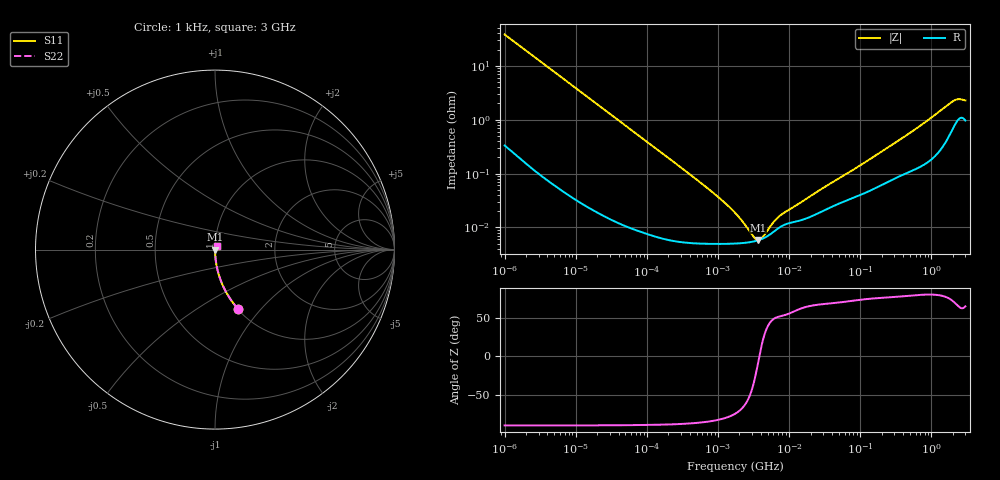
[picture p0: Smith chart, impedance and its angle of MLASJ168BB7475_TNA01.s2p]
! MLASJ168BB7475_TNA01  S-PARAMETER MODEL  ( Standard Model )
! Model Generated by TAIYO YUDEN Corporation (http://www.ty-top.com)
! Version 1.0
! TAIYO YUDEN Control No. 220601
! Copyright(c) 2014 TAIYO YUDEN CO.,LTD. All Rights Reserved.
! Product Description (link to TY-COMPAS)
! https://ds.yuden.co.jp/TYCOMPAS/or/detail?pn=MLASJ168BB7475KTNA01&u=M
! Products Name : Multilayer Ceramic Capacitors
! Characteristics :
!  Capacitance : 4.7 [uF] , Rated Voltage : 6.3 [V] , TCC : X7R
!  Case Size : 1.6 x 0.8 / 0.063 x 0.031 [mm/inch] , Thickness : 0.8 / 0.031 [mm/inch]
!  (Conditions: Temperature = 25 [degC] , DC Bias Voltage = 0 [V])
! External Node Assignments :
!  1  o---| |---o  2
! GND o---------o GND
! Frequency Range : 1kHz  -  3GHz  [ 401 STEP ]
# MHZ S RI R 50
! Freq[MHz].  S11 Real  S11 Imag  S21 Real  S21 Imag  S12 Real  S12 Imag  S22 Real  S22 Imag
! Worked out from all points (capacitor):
!   401 points, 1 kHz to 3 GHz, reference 50 ohm
!   read as one part in series: C = 4.16 uF near 1.077 kHz
!   lowest |Z| = 5.82 mohm at 3.651 MHz (marker M1)
!   series resonance near 3.805 MHz, so ESL is about 420 pH
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0.001  0.1293 -0.3313  0.8707 0.3313  0.8707 0.3313  0.1293 -0.3313
0.001685  0.0507 -0.2153  0.9493 0.2153  0.9493 0.2153  0.0507 -0.2153
0.00306  0.0164 -0.1233  0.9836 0.1233  0.9836 0.1233  0.0164 -0.1233
0.005768  0.00495 -0.0664  0.995 0.0664  0.995 0.0664  0.00495 -0.0664
0.01216  0.00128 -0.0317  0.9987 0.0317  0.9987 0.0317  0.00128 -0.0317
0.147855  7.14e-05 -0.00264  0.9999 0.00264  0.9999 0.00264  7.14e-05 -0.00264
0.791611  4.97e-05 -0.000475  1 0.000475  1 0.000475  4.97e-05 -0.000475
1.238299  4.96e-05 -0.000284  1 0.000284  1 0.000284  4.96e-05 -0.000284
1.732051  5.02e-05 -0.00018  0.9999 0.00018  0.9999 0.00018  5.02e-05 -0.00018
2.422679  5.18e-05 -9.7e-05  0.9999 9.7e-05  0.9999 9.7e-05  5.18e-05 -9.7e-05
2.610246  5.24e-05 -8.02e-05  0.9999 8.02e-05  0.9999 8.02e-05  5.24e-05 -8.02e-05
3.651041  5.75e-05 -8.57e-06  0.9999 8.57e-06  0.9999 8.57e-06  5.75e-05 -8.57e-06
4.919932  6.86e-05 5.33e-05  0.9999 -5.33e-05  0.9999 -5.33e-05  6.86e-05 5.33e-05
5.30084  7.31e-05 6.86e-05  0.9999 -6.86e-05  0.9999 -6.86e-05  7.31e-05 6.86e-05
6.881678  9.43e-05 0.000118  0.9999 -0.000118  0.9999 -0.000118  9.43e-05 0.000118
7.988506  0.000107 0.000141  0.9999 -0.000141  0.9999 -0.000141  0.000107 0.000141
21.06097  0.000163 0.000368  0.9998 -0.000368  0.9998 -0.000368  0.000163 0.000368
256.0921  0.000733 0.00309  0.9993 -0.00309  0.9993 -0.00309  0.000733 0.00309
650.4536  0.00132 0.00712  0.9987 -0.00712  0.9987 -0.00712  0.00132 0.00712
1990.675  0.0071 0.0205  0.9929 -0.0205  0.9929 -0.0205  0.0071 0.0205
2398.636  0.0105 0.0214  0.9895 -0.0214  0.9895 -0.0214  0.0105 0.0214
3000  0.00994 0.0203  0.9901 -0.0203  0.9901 -0.0203  0.00994 0.0203
